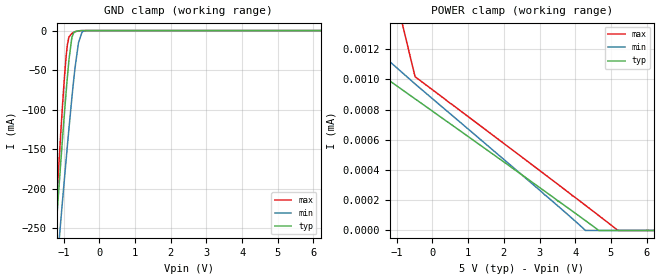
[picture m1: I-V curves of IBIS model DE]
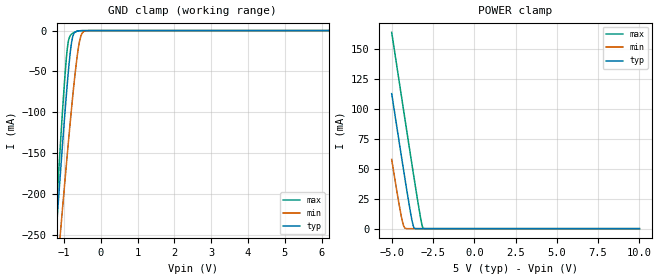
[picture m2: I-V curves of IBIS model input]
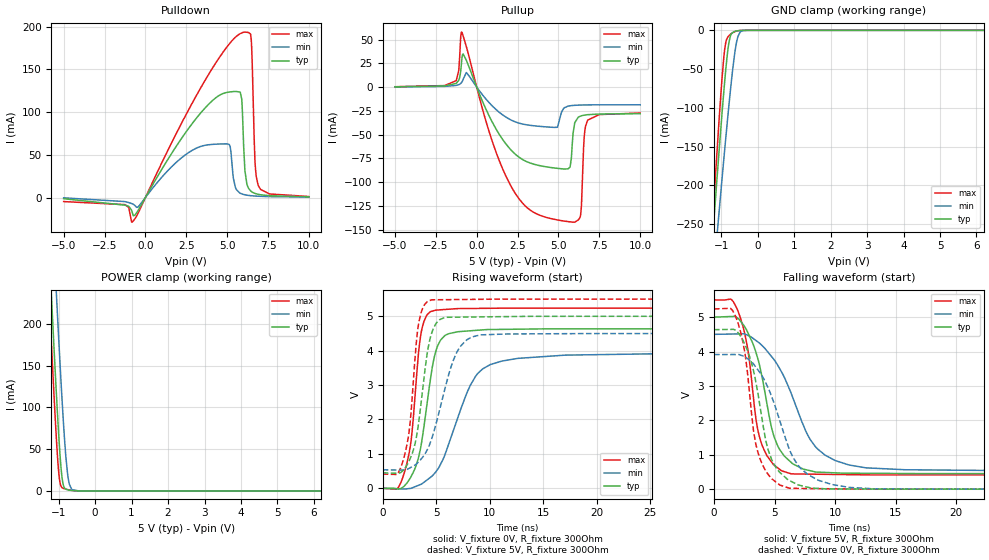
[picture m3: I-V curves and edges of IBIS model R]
|Texas Instruments Incorporated
|THVD1505 Bus-Polarity Correcting RS-485 Transceiver With IEC-ESD Protection
[IBIS Ver]   4.1
[File name]   thvd1505.ibs
[Date]   12/07/2018
[File Rev]   1.0
[Source]
| Texas Instruments Incorporated.
| Analog-eLab Design Center, HPA
| 12500 TI Blvd
| Dallas, TX -75243
[Notes]   Revision History:
| Rev 1.0: 12/07/2018
| - Initial version of the model
| - Model generated from simulations in SPECTRE
| - Warnings regarding combined Non-monotonicity of various models
|   have been reviewed and considered minor and can be ignored.
| - Connect 1uF capacitor at the common mode node for "diffout" model.
| - C_comp although listed in numerical order of value are
|   obtained from varying PVT conditions. For PVT conditions for
|   each specific value refer the buffer description under
|   respective [Model]. IBIS model user is responsible for using
|   appropriate C_comp to simulate for Signal Integrity.
[Disclaimer]
| This model is designed as an aid for customers of Texas Instruments.
| TI and its licensors and suppliers make no warranties, either expressed
| or implied, with respect to this  model, including the warranties of
| merchantability or fitness for a particular purpose. The model is
| provided solely on an "as is" basis. The entire risk as to its quality
| and performance is with the customer.
| This model is subject to change without notice. Texas Instruments
| Incorporated is not responsible for updating this model.
[Copyright]
(C) Copyright 2018 Texas Instruments Incorporated.All rights reserved.
|  Component THVD1505D 8-pin SOIC - D package
|  Part # THVD1505D
[Component]   THVD1505D
[Manufacturer]  TI
[Package]   |8 SOIC - D package
|   typ   min   max
R_pkg   0.05   0.04   0.06
L_pkg   1.0nH   0.8nH   1.2nH
C_pkg   0.2pF   0.16pF   0.24pF
[Pin]  signal_name  model_name   R_pin   L_pin   C_pin
1   R   R   NA   NA   NA
2   _RE   input   NA   NA   NA
3   DE   DE   NA   NA   NA
4   D   input   NA   NA   NA
5   GND   gnd   NA   NA   NA
6   A   diffout   NA   NA   NA
7   B   diffout   NA   NA   NA
8   VCC   power   NA   NA   NA
[Diff_pin]   inv_pin   vdiff   tdelay_typ   tdelay_min   tdelay_max
6   7   0.100   NA   NA   NA
| Models and submodels in the file (4): DE (Input), input (Input), R (3-state), diffout (I/O)
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|   DE Model
[Model]   DE
Model_type   Input
Vinl = 0.8
Vinh = 2
|   typ   min   max
C_comp   2.247pF   2.186pF   2.332pF
| Where Nom  PVT is Nominal Process, 5.0V, 25C
|   Fast PVT is Strong Process,  5.5V, -40C
|   Slow PVT is Weak Process,   4.5V, 150C
[Voltage Range]   5   4.5   5.5
|Junction Temperature
[Temperature Range]   25   150   -40
[Power Clamp Reference]   5   4.5   5.5
[GND Clamp Reference]   0   0   0
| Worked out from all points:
|   GND clamp passes 1 mA (typ) near -0.65 V on its own axis
[GND Clamp]
|   Voltage   I(typ)   I(min)   I(max)
-3.5V     -1.774A    -1.581A    -2.051A
-1.28V    -291.9mA   -346.6mA   -277.7mA
-1.076V   -163.2mA   -238.1mA   -125.4mA
-980mV    -105.5mA   -188.2mA   -60.51mA
-920mV    -71.66mA   -157.7mA   -27.64mA
-860mV    -41.06mA   -127.9mA   -9.56mA
-776mV    -10.64mA   -87.86mA   -3.758mA
-692mV    -1.735mA   -51.25mA   -1.576mA
-584mV    -284.2uA   -15.24mA   -296uA
-488mV    -51.93uA   -2.192mA   -42.77uA
-392mV    -7.53uA    -207.4uA   -4.292uA
8.5V      0A         0A         0A
[POWER Clamp]
|   Voltage   I(typ)   I(min)   I(max)
-3.5V     4.624uA    1.653uA    29.39mA
-3.188V   1.322uA    1.536uA    4.469mA
-2.984V   1.288uA    1.489uA    3.464uA
-488mV    870.7nA    969.3nA    1.017uA
2.608V    350.7nA    346.8nA    467.2nA
4.288V    64.77nA    46.39pA    166nA
4.66V     155.3pA    0A         98.63nA
5.212V    0A         0A         0A
8.5V      0A         0A         0A
|   input Model
[Model]   input
Model_type   Input
Vinl = 0.8
Vinh = 2
|   typ   min   max
C_comp   2.247pF   2.186pF   2.332pF
| Where Nom  PVT is Nominal Process, 5.0V, 25C
|   Fast PVT is Strong Process,  5.5V, -40C
|   Slow PVT is Weak Process,   4.5V, 150C
[Voltage Range]   5   4.5   5.5
|Junction Temperature
[Temperature Range]   25   150   -40
[Power Clamp Reference]   5   4.5   5.5
[GND Clamp Reference]   0   0   0
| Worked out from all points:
|   GND clamp passes 1 mA (typ) near -0.66 V on its own axis
|   POWER clamp passes 1 mA (typ) near -3.66 V on its own axis
[GND Clamp]
|   Voltage   I(typ)   I(min)   I(max)
-5V       -2.789A    -2.427A    -3.264A
-1.235V   -263.1mA   -322.4mA   -243.3mA
-1.145V   -206mA     -274.5mA   -175.7mA
-1.07V    -159.5mA   -234.9mA   -121.1mA
-980mV    -105.5mA   -188.2mA   -60.51mA
-905mV    -63.61mA   -150.2mA   -21.4mA
-860mV    -41.06mA   -127.9mA   -9.56mA
-785mV    -12.82mA   -92.02mA   -4.076mA
-650mV    -835.2uA   -35.2mA    -894.6uA
-545mV    -146.3uA   -7.66mA    -140.2uA
-410mV    -11.97uA   -325uA     -7.926uA
10V       0A         0A         0A
[POWER Clamp]
|   Voltage   I(typ)   I(min)   I(max)
-5V       112.7mA    57.75mA    163.8mA
-4.55V    72.57mA    20.12mA    123.1mA
-4.31V    51.43mA    3.786mA    101.5mA
-4.16V    38.4mA     210.5uA    88.05mA
-3.875V   14.6mA     182.7nA    62.59mA
-3.725V   3.965mA    29.27nA    49.3mA
-3.665V   1.246mA    24.26nA    44.02mA
-3.605V   208.1uA    20.95nA    38.76mA
-3.26V    0A         6.508nA    9.736mA
-3.14V    0A         2.405nA    1.842mA
-3.08V    0A         507.5pA    242.3uA
10V       0A         0A         0A
|   R Model
[Model]   R
Model_type   3-state
Polarity   Non-Inverting
Vmeas = 2.5
Vref = 0
Cref = 2pF
Rref = 100000
|   typ   min   max
C_comp   3.781pF   3.678pF   3.870pF
| Where Nom  PVT is Nominal Process, 5.0V, 25C
|   Fast PVT is Strong Process,  5.5V, -40C
|   Slow PVT is Weak Process,   4.5V, 150C
[Voltage Range]   5   4.5   5.5
|Junction Temperature
[Temperature Range]   25   150   -40
[Pullup Reference]   5   4.5   5.5
[Pulldown Reference]   0   0   0
[Power Clamp Reference]   5   4.5   5.5
[GND Clamp Reference]   0   0   0
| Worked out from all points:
|   slope of the pulldown table from 0 to 0.75 V, typ, clamps not added: 30.1 ohm
|   slope of the pullup table from 0 to 0.75 V, typ, clamps not added: 25 ohm
|   GND clamp passes 1 mA (typ) near -0.60 V on its own axis
|   POWER clamp passes 1 mA (typ) near -0.71 V on its own axis
|   falling waveform, V_fixture 5V, R_fixture 300Ohm: 20-80 % time 1.78ns typ, 3.11ns min, 1.27ns max; typ from 5 V to 0.451 V
|   rising waveform, V_fixture 0V, R_fixture 300Ohm: 20-80 % time 1.38ns typ, 2.9ns min, 959ps max; typ from 0 V to 4.64 V
|   rising waveform, V_fixture 5V, R_fixture 300Ohm: 20-80 % time 1.18ns typ, 2.14ns min, 862ps max; typ from 0.451 V to 5 V
|   falling waveform, V_fixture 0V, R_fixture 300Ohm: 20-80 % time 1.63ns typ, 2.56ns min, 1.22ns max; typ from 4.64 V to 0 V
[Pulldown]
|   Voltage   I(typ)   I(min)   I(max)
-5V       -1.413mA   -385.7uA   -4.759mA
-815mV    -16.82mA   -7.252mA   -28.82mA
4.735V    121.7mA    62.75mA    169.7mA
5.17V     123.6mA    60.36mA    180.7mA
5.38V     124mA      22.52mA    185.3mA
5.8V      123.2mA    5.053mA    191.8mA
5.905V    111.3mA    4.162mA    192.8mA
6.085V    31.62mA    3.183mA    193.6mA
6.475V    7.096mA    2.097mA    184.3mA
6.7V      4.806mA    1.749mA    43.21mA
6.895V    3.745mA    1.528mA    14.5mA
10V       816.9uA    503.2uA    1.18mA
[GND Clamp]
|   Voltage   I(typ)   I(min)   I(max)
-5V       -2.812A    -2.47A     -3.273A
-1.235V   -266.2mA   -328.5mA   -245mA
-1.145V   -208.8mA   -279.7mA   -177.3mA
-1.07V    -161.8mA   -239.5mA   -122.8mA
-980mV    -107.5mA   -192mA     -62.42mA
-920mV    -73.47mA   -161mA     -30.09mA
-860mV    -42.74mA   -130.7mA   -12.71mA
-785mV    -14.47mA   -94.16mA   -6.709mA
-635mV    -1.515mA   -31.07mA   -1.789mA
-545mV    -512.1uA   -8.21mA    -558.8uA
-395mV    -39.69uA   -313.1uA   -27.5uA
10V       0A         0A         0A
[Pullup]
|   Voltage   I(typ)   I(min)   I(max)
-5V       294uA      201.9uA    371.4uA
-1.25V    3.885mA    1.772mA    6.733mA
-920mV    27.3mA     4.943mA    57.9mA
910mV     -35.48mA   -19.11mA   -54.94mA
2.215V    -68.29mA   -35.6mA    -107.9mA
4.915V    -85.5mA    -42.32mA   -139.8mA
5.575V    -86.08mA   -20.15mA   -141.6mA
5.845V    -59.81mA   -19.41mA   -142.2mA
6.355V    -30.52mA   -18.92mA   -134.9mA
6.58V     -29.54mA   -18.82mA   -51.42mA
6.79V     -29.05mA   -18.76mA   -34.78mA
10V       -28mA      -18.64mA   -27.28mA
[POWER Clamp]
|   Voltage   I(typ)   I(min)   I(max)
-5V       3.962A     4.069A     3.914A
-1.415V   433.6mA    556.6mA    376.6mA
-1.25V    279.9mA    403.4mA    222.3mA
-1.175V   212.2mA    335.1mA    154.8mA
-1.07V    121.7mA    242.1mA    67.41mA
-980mV    53.58mA    165.9mA    14.39mA
-920mV    20.46mA    118.4mA    4.493mA
-860mV    5.309mA    75.14mA    2.857mA
-800mV    1.996mA    39.28mA    2.076mA
-710mV    969.4uA    8.417mA    1.17mA
-455mV    33.66uA    93.87uA    20.17uA
10V       0A         0A         0A
[Ramp]
R_load = 300
|   typ   min   max
dV/dt_r   2.78147/1.3731e-09   2.34775/2.8694e-09   3.14208/9.56339e-10
dV/dt_f   2.72918/1.76898e-09   2.37774/3.09049e-09   3.05203/1.26458e-09
[Falling Waveform]
V_fixture = 5V
V_fixture_min = 4.5V
V_fixture_max = 5.5V
R_fixture = 300Ohm
C_fixture = 0F
|   Time   V(typ)   V(min)   V(max)
0s        5V         4.5V       5.5V
1.594ns   5.021V     4.51V      5.451V
2.685ns   4.631V     4.488V     4.266V
3.47ns    3.969V     4.319V     2.023V
3.936ns   3.311V     4.186V     1.312V
4.968ns   1.513V     3.759V     697.8mV
6.38ns    775mV      2.775V     444.4mV
8.558ns   495.5mV    1.165V     434mV
12.55ns   461.5mV    619.5mV    415.8mV
100ns     451.4mV    537.1mV    413.3mV
[Rising Waveform]
V_fixture = 0V
V_fixture_min = 0V
V_fixture_max = 0V
R_fixture = 300Ohm
C_fixture = 0F
|   Time   V(typ)   V(min)   V(max)
0s        -39.05nV   250.9nV    -737.6pV
1.862ns   26.07mV    -17.12mV   298.7mV
2.589ns   304mV      -2.724mV   1.236V
3.045ns   598mV      48.4mV     2.76V
3.704ns   1.468V     138.2mV    4.682V
4.92ns    3.929V     458.8mV    5.175V
5.937ns   4.462V     1.077V     5.2V
8.7ns     4.59V      3.261V     5.228V
12.65ns   4.624V     3.776V     5.236V
100ns     4.636V     3.913V     5.237V
[Rising Waveform]
V_fixture = 5V
V_fixture_min = 4.5V
V_fixture_max = 5.5V
R_fixture = 300Ohm
C_fixture = 0F
|   Time   V(typ)   V(min)   V(max)
0s        451.4mV    537.1mV    413.3mV
1.647ns   453.8mV    530.3mV    568.9mV
2.393ns   747.2mV    567mV      1.482V
2.775ns   1.024V     633.1mV    2.712V
3.16ns    1.504V     710.5mV    4.287V
3.432ns   2.077V     790.5mV    4.902V
4.555ns   4.485V     1.416V     5.476V
6.849ns   4.973V     3.9V       5.486V
9.23ns    4.982V     4.46V      5.493V
100ns     5V         4.5V       5.5V
[Falling Waveform]
|Gnd
V_fixture = 0V
V_fixture_min = 0V
V_fixture_max = 0V
R_fixture = 300Ohm
C_fixture = 0F
|   Time   V(typ)   V(min)   V(max)
0s        4.636V     3.913V     5.237V
1.529ns   4.645V     3.914V     5.197V
2.357ns   4.354V     3.877V     4.322V
3.258ns   3.449V     3.642V     1.713V
3.704ns   2.616V     3.43V      981.4mV
4.777ns   845.5mV    2.675V     298.9mV
6.245ns   248.5mV    1.138V     25.18mV
8.558ns   21.98mV    269.3mV    15.66mV
13.17ns   3.702mV    11.02mV    761.9uV
100ns     -26.23nV   218.3nV    12.38nV
